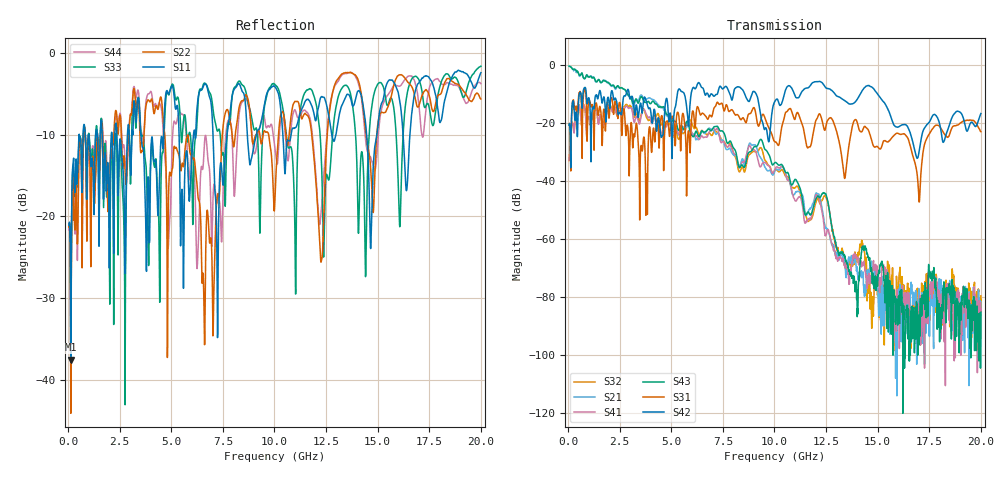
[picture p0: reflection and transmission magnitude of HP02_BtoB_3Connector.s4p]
# MHz S MA R 50.00
! FREQ  S11  S12  S13  S14
!  S21  S22  S23  S24
!  S31  S32  S33  S34
!  S41  S42  S43  S44
!  MAG  ANG  MAG  ANG  MAG  ANG  MAG  ANG
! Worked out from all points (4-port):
!   1996 points, 50 MHz to 20 GHz, reference 50 ohm
!   strongest paths, dB at 50 MHz, 5.04 GHz, 10.03 GHz, 15.02 GHz, 20 GHz:
!     S42: -20.9, -32.3, -12.5, -10.3, -16.8
!     S31: -20.9, -17.9, -26.6, -28.4, -23.1
!     S43: -0.5, -18.7, -33.7, -72.3, -85.2
!     S41: -32.9, -21.6, -35.8, -71.2, -85.0
!     S21: -0.5, -21.1, -36.4, -79.7, -88.6
!     S32: -33.0, -23.8, -36.2, -77.7, -79.6
!   lowest |S11| = -37.5 dB at 130 MHz (marker M1), VSWR 1.03, Z = 51.3 - j0.17 ohm
!   |S11| at or under -10 dB: 3.526 GHz to 4.627 GHz (1.1 GHz wide, 27 % of centre); 5.378 GHz to 6.075 GHz (697.8 MHz wide, 12.2 % of centre); 7.022 GHz to 7.701 GHz (679.7 MHz wide, 9.23 % of centre)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
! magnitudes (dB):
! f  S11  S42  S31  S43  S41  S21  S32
! 50 MHz  -21.1  -20.9  -20.9  -0.5  -32.9  -0.5  -33.0
! 130 MHz  -37.5  -35.5  -36.6  -0.8  -24.5  -0.8  -24.5
! 7.18 GHz  -19.9  -10.3  -13.6  -21.2  -22.2  -24.0  -23.0
! 12.45 GHz  -5.7  -7.6  -22.5  -44.3  -58.8  -55.7  -45.0
! 13.97 GHz  -5.1  -12.3  -19.2  -76.0  -66.9  -71.0  -67.5
! 17 GHz  -3.7  -30.3  -46.4  -96.5  -83.9  -77.1  -82.0
! 20 GHz  -2.4  -16.8  -23.1  -85.2  -85.0  -88.6  -79.6
